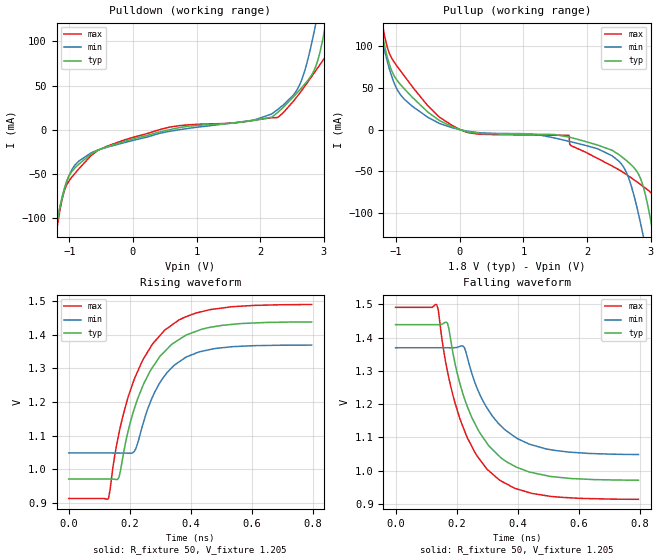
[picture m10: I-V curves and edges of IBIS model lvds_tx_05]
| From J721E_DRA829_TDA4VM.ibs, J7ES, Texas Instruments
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|   MODEL lvds_tx_05
[Model] lvds_tx_05
Model_type Output
C_comp 1.579p 1.586p 1.519p
Vmeas = 1.2
Vref = 1.2V
Rref = 50
Cref = 0.5pF
[Model Spec]
[Temperature Range]  40 150 -40
[Voltage Range] 1.8 1.62 1.98
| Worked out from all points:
|   slope of the pulldown table from 0 to 0.27 V, typ, clamps not added: 55 ohm
|   slope of the pullup table from 0 to 0.27 V, typ, clamps not added: 62.9 ohm
|   rising waveform, R_fixture 50, V_fixture 1.205: 20-80 % time 125ps typ, 104ps min, 128ps max; typ from 0.971 V to 1.44 V
|   falling waveform, R_fixture 50, V_fixture 1.205: 20-80 % time 126ps typ, 128ps min, 124ps max; typ from 1.44 V to 0.971 V
[Pulldown]
-1.715V   -358.6mA   -310.7mA   -422.9mA
-1.208V   -111.4mA   -107.4mA   -119.2mA
-1.102V   -73.28mA   -74.33mA   -75.69mA
-1.007V   -52.86mA   -52.61mA   -58.33mA
-552.1mV  -23.11mA   -22.96mA   -23.35mA
574.5mV   0A         -1.742mA   2.937mA
2.277V    19.58mA    22.94mA    13.8mA
2.631V    45.78mA    52.47mA    42.29mA
2.864V    69.77mA    116.1mA    65.71mA
3.017V    114.3mA    174.1mA    81.87mA
3.175V    184mA      238.8mA    118.2mA
3.514V    352.3mA    380.7mA    306.3mA
[Pullup]
-1.714V   352.3mA    305.1mA    416.6mA
-1.27V    136mA      125.5mA    152.9mA
-989.5mV  59.78mA    49.12mA    76.69mA
-503.1mV  21.28mA    14.99mA    28.81mA
120.9mV   -2.53mA    -1.802mA   -3.347mA
1.718V    -8.809mA   -13.93mA   -6.729mA
2.394V    -24.66mA   -31.28mA   -43.54mA
2.648V    -38.9mA    -56.68mA   -55.2mA
2.876V    -66.13mA   -124.4mA   -67.63mA
3.045V    -127.1mA   -190mA     -79.17mA
3.188V    -193.5mA   -248.7mA   -122.4mA
3.515V    -358.6mA   -386.4mA   -311.5mA
[Ramp]
dV/dt_r .281/125.468p .193/104.532p .347/128.093p
dV/dt_f .281/126.414p .193/127.747p .347/124.452p
[Rising Waveform]
R_fixture = 50
V_fixture = 1.205
V_fixture_min = 1.209
V_fixture_max = 1.202
0s        970.8mV    1.048V     912.8mV
130ps     970.5mV    1.048V     911.9mV
165ps     976.9mV    1.048V     1.109V
195ps     1.115V     1.048V     1.216V
220ps     1.195V     1.062V     1.279V
245ps     1.254V     1.14V      1.329V
315ps     1.352V     1.279V     1.415V
385ps     1.4V       1.334V     1.455V
475ps     1.425V     1.359V     1.477V
795ps     1.439V     1.37V      1.491V
[Falling Waveform]
R_fixture = 50
V_fixture = 1.205
V_fixture_min = 1.209
V_fixture_max = 1.202
0s        1.439V     1.37V      1.491V
135ps     1.439V     1.37V      1.499V
170ps     1.444V     1.37V      1.298V
210ps     1.264V     1.374V     1.157V
225ps     1.218V     1.371V     1.121V
270ps     1.123V     1.241V     1.04V
340ps     1.043V     1.139V     971.4mV
400ps     1.008V     1.095V     943.8mV
495ps     984.2mV    1.065V     923.9mV
795ps     970.8mV    1.048V     913.2mV
